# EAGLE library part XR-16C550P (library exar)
UART/FIFO
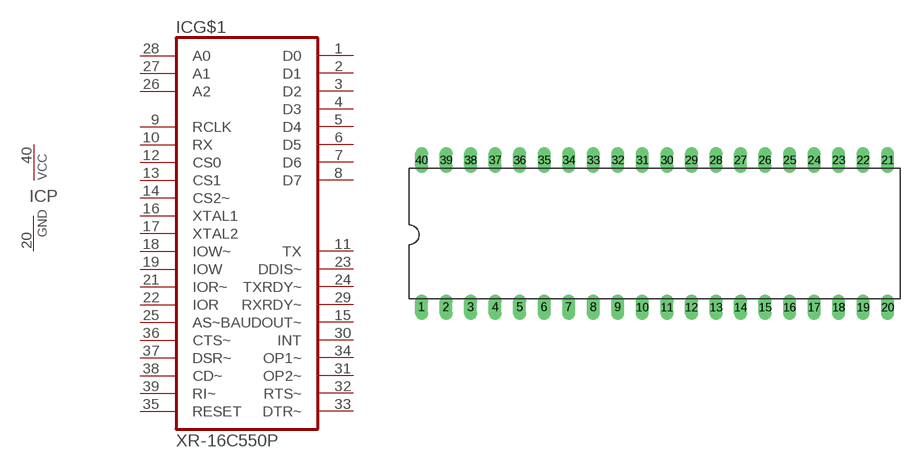
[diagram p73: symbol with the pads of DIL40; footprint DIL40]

Designator prefix IC; gates G$1=16C550 P=PWRN

## XR-16C550P (MPN: ST16C450CP40; OC_FARNELL: 1294801; OC_NEWARK: 24R1445)  [DIL40]
1  G$1:D0
2  G$1:D1
3  G$1:D2
4  G$1:D3
5  G$1:D4
6  G$1:D5
7  G$1:D6
8  G$1:D7
9  G$1:RCLK  in
10  G$1:RX  in
11  G$1:TX  out
12  G$1:CS0  in
13  G$1:CS1  in
14  G$1:CS2~  in
15  G$1:BAUDOUT~  out
16  G$1:XTAL1  in
17  G$1:XTAL2  in
18  G$1:IOW~  in
19  G$1:IOW  in
20  P:GND  pwr
21  G$1:IOR~  in
22  G$1:IOR  in
23  G$1:DDIS~  out
24  G$1:TXRDY~  out
25  G$1:AS~  in
26  G$1:A2  in
27  G$1:A1  in
28  G$1:A0  in
29  G$1:RXRDY~  out
30  G$1:INT  out
31  G$1:OP2~  out
32  G$1:RTS~  out
33  G$1:DTR~  out
34  G$1:OP1~  out
35  G$1:RESET  in
36  G$1:CTS~  in
37  G$1:DSR~  in
38  G$1:CD~  in
39  G$1:RI~  in
40  P:VCC  pwr

## Footprint DIL40 (pad centres in mm)
Dual In Line Package
drill 0.813 long: 1 -24.13,-7.62; 2 -21.59,-7.62; 3 -19.05,-7.62; 4 -16.51,-7.62; 5 -13.97,-7.62; 6 -11.43,-7.62; 7 -8.89,-7.62; 8 -6.35,-7.62; 9 -3.81,-7.62; 10 -1.27,-7.62; 11 1.27,-7.62; 12 3.81,-7.62; 13 6.35,-7.62; 14 8.89,-7.62; 15 11.43,-7.62; 16 13.97,-7.62; 17 16.51,-7.62; 18 19.05,-7.62; 19 21.59,-7.62; 20 24.13,-7.62; 21 24.13,7.62; 22 21.59,7.62; 23 19.05,7.62; 24 16.51,7.62; 25 13.97,7.62; 26 11.43,7.62; 27 8.89,7.62; 28 6.35,7.62; 29 3.81,7.62; 30 1.27,7.62; 31 -1.27,7.62; 32 -3.81,7.62; 33 -6.35,7.62; 34 -8.89,7.62; 35 -11.43,7.62; 36 -13.97,7.62; 37 -16.51,7.62; 38 -19.05,7.62; 39 -21.59,7.62; 40 -24.13,7.62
